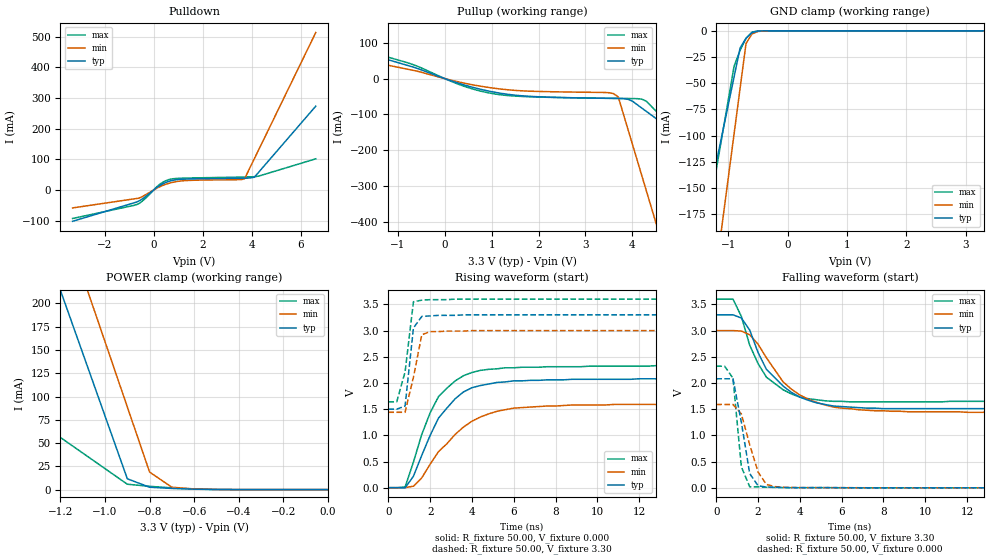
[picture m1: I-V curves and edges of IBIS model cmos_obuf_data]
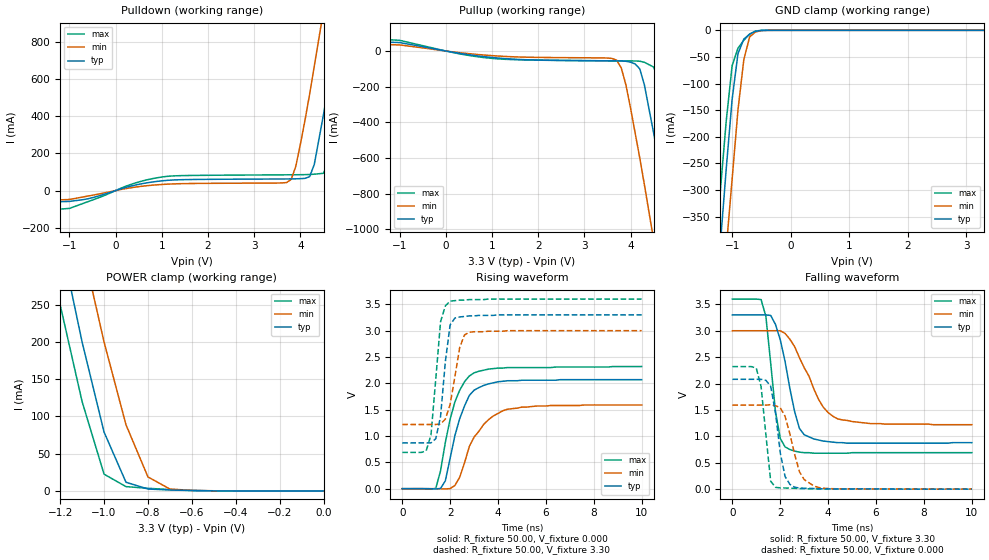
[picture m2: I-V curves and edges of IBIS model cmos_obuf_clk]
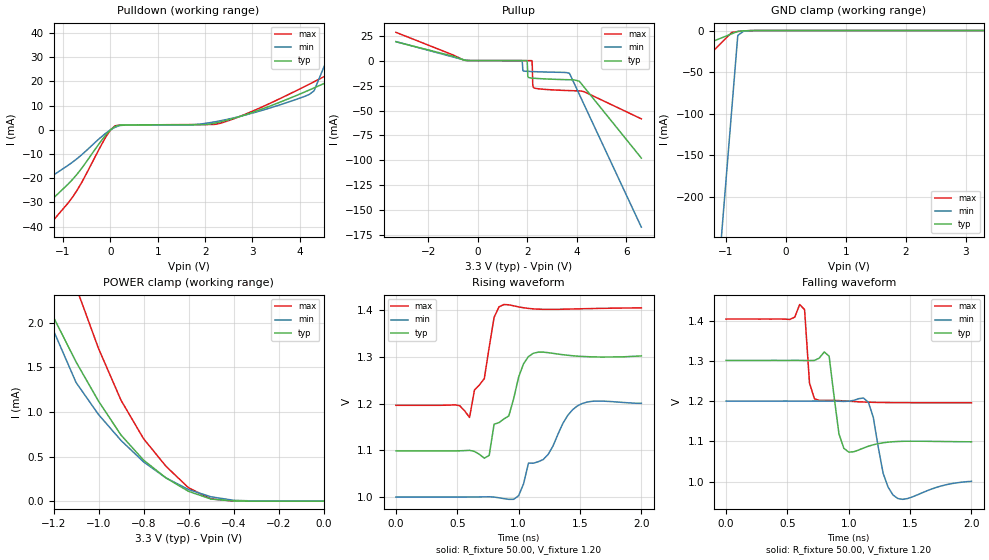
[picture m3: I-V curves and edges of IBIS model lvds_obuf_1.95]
| TEXAS INSTRUMENTS INCORPORATED
| High Performance Analog Group
| IBIS Model for ADS5545/46/47/25/27 series of A/D converters
| This file provides unique models under the [Model Selector] for each
| load condition.
| For operation at a specific load condition, select the appropriate model
|after each [Model Selector] keyword.
[IBIS ver]   3.2
[File name]   ads554x.ibs
[File Rev]   0
[Date]   17 Jul 2006
[Source]   Data created from TI-SPICE simulations
[Disclaimer] Property of Texas Instruments Incorporated.
   Unauthorized reproduction and/or distribution is strictly
   protected under copyright law. Created 2006, (C) Copyright
   2006, Texas Instruments Incorporated, All Rights Reserved
   UNLESS THERE IS A SIGNED, WRITTEN AGREEMENT TO THE CONTRARY,
   TEXAS INSTRUMENTS (TI) IS PROVIDING THE IBIS MODELS AND
   WITHOUT ANY WARRANTY, EXPRESSED OR IMPLIED. TI assumes no
   liability for: 1) the accuracy of the IBIS models provided to
   your company; 2) the proper functioning of these IBIS Models
   in your design or for any resulting applications; or 3)
   infringement of patents, copyrights or intellectual property
   rights resulting from your use of these IBIS models. TI
   provides IBIS Models as a service to our customers. You and
   your company shall not distribute, sell or give these models
   to anyone else without prior written permission from TI.
   TI reserves the right to make changes to our products or
   to discontinue any semiconductor product or service
   without notice, and advises our customers to obtain the
   latest version of relevant information to verify, before
   placing orders, that the information being relied on is
   current.
   Please be aware that your receipt and use of the IBIS
   information provided shall serve as acceptance of these
   terms and conditions.  If you do not accept these terms,
   you should return or destroy the IBIS models and any
   other accompanying information immediately.
[Notes]   This file contains IBIS Model of various buffers of
   ADS5545/46/47/25/27 series of A/D converters
[Copyright]   Property of Texas Instruments Incorporated. Unauthorised
   reproduction and/or distribution is strictly prohibited. This
   product is protected under copyright law and trade secret law
   as an unpublished work. Created 2000,(C) Copyright 2000,Texas
   Instruments Inc., All Rights Reserved.These commodities are
   under the U.S. Government distribution license control.As
   such,they are not to be re-exported without the prior approval
   of the U.S. Department of Commerce.
|   Component ADS554X
[Component]   ADS554X
[Manufacturer]   Texas Instruments
[Package]
| variable   typ   min   max
R_pkg   0.438   0.327   0.55
L_pkg   1.442nH   1.022nH   1.87nH
C_pkg   0.13pF   0.08390pF   0.201pF
[Pin]   signal_name   model_name   R_pin   L_pin   C_pin
|   (ohms)   (nH)   (pF)
1   DRGND   GND
2   DRVDD   POWER
3   OVR   cmos_obuf_data
4   CLKOUTM   clockoutm
5   CLKOUTP   clockoutp
|6   DFS   dummy
|7   OE   dummy
8   AVDD   POWER
9   AGND   POWER
10   CLKP   input
11   CLKM   input
12   AGND   GND
|13   VCMOUT / REFIN   dummy
14   AGND   GND
|15   INP   dummy
|16   INM   dummy
17   AGND   GND
18   AVDD   POWER
19   AGND   GND
20   AVDD   POWER
|21   IREF   dummy
22   AVDD   POWER
|23   MODE   dummy
24   AVDD   POWER
25   AGND   GND
26   AVDD   POWER
|27   SEN   dummy
|28   SDATA   dummy
|29   SCLK   dummy
|30   RESET   dummy
31   NC   NC
32   NC   NC
33   D0_D1M/D0   dataoutput
34   D0_D1P/D1   dataoutput
35   DRVDD   POWER
36   DRGND   GND
37   D2_D3M/D2   dataoutput
38   D2_D3P/D3   dataoutput
39   D4_D5M/D4   dataoutput
40   D4_D5P/D5   dataoutput
41   D6_D7M/D6   dataoutput
42   D6_D7P/D7   dataoutput
43   D8_D9M/D8   dataoutput
44   D8_D9P/D9   dataoutput
45   D10_D11M/D10   dataoutput
46   D10_D11P/D11   dataoutput
47   D12_D13M/D12   dataoutput
48   D12_D13P/D13   dataoutput
[Diff Pin]   inv_pin   vdiff   tdelay_typ   tdelay_min   tdelay_max
  4   5   350mV   0   0   0
  10   11   350mV   0   0   0
  34   33   350mV   0   0   0
  38   37   350mV   0   0   0
  40   39   350mV   0   0   0
  42   41   350mV   0   0   0
  44   43   350mV   0   0   0
  46   45   350mV   0   0   0
  48   47   350mV   0   0   0
[Series Pin Mapping]  pin_2   model_name   function_table_group
  4   5   series_res_166   1
  4   5   series_res_200   2
  4   5   series_res_333   3
  10   11   series_cap
  34   33   series_res_166   1
  34   33   series_res_200   2
  34   33   series_res_333   3
  38   37   series_res_166   1
  38   37   series_res_200   2
  38   37   series_res_333   3
  40   39   series_res_166   1
  40   39   series_res_200   2
  40   39   series_res_333   3
  42   41   series_res_166   1
  42   41   series_res_200   2
  42   41   series_res_333   3
  44   43   series_res_166   1
  44   43   series_res_200   2
  44   43   series_res_333   3
  46   45   series_res_166   1
  46   45   series_res_200   2
  46   45   series_res_333   3
  48   47   series_res_166   1
  48   47   series_res_200   2
  48   47   series_res_333   3
[Series Switch Groups]
| Following represent all possible switching combinations for 5 series elements
Off 1 2 3  /
Off 1 2 /
Off 2 3 /
Off 1 3 /
Off 1 /
Off 2 /
Off 3 /
On 1 2 3  /
[Model Selector] clockoutp
|The clock output can be in lvds mode or cmos mode. In lvds mode the
|clock signal ia a differential signal between pins CLKOUTP and CLKOUTM
|and in cmos mode its a single ended signal at pin CLKOUTP only.
|Note that the model for cmos buffer is different for data and clock output
|buffers whereas the model for the lvds buffer is the same
|  Model name   Description
cmos_obuf_clk   CMOS tri-state buffer
lvds_obuf_1.95   LVDS tri-state buffer with current setting 1.95mA
lvds_obuf_2.5   LVDS tri-state buffer with current setting 2.5mA
lvds_obuf_3.5   LVDS tri-state buffer with current setting 3.5mA
lvds_obuf_3.9   LVDS tri-state buffer with current setting 3.9mA
lvds_obuf_4.5   LVDS tri-state buffer with current setting 4.5mA
lvds_obuf_5.0   LVDS tri-state buffer with current setting 5.0mA
lvds_obuf_7.0   LVDS tri-state buffer with current setting 7.0mA
lvds_obuf_9.0   LVDS tri-state buffer with current setting 9.0mA
[Model Selector] clockoutm
|When the clock is output in the cmos mode, CLOCKOUTM is disabled. In the
|lvds mode the clock output is a differential signal between pins CLKOUTP
|and CLKOUTM.
|  Model name   Description
lvds_obuf_1.95   LVDS tri-state buffer with current setting 1.95mA
lvds_obuf_2.5   LVDS tri-state buffer with current setting 2.5mA
lvds_obuf_3.5   LVDS tri-state buffer with current setting 3.5mA
lvds_obuf_3.9   LVDS tri-state buffer with current setting 3.9mA
lvds_obuf_4.5   LVDS tri-state buffer with current setting 4.5mA
lvds_obuf_5.0   LVDS tri-state buffer with current setting 5.0mA
lvds_obuf_7.0   LVDS tri-state buffer with current setting 7.0mA
lvds_obuf_9.0   LVDS tri-state buffer with current setting 9.0mA
[Model Selector] dataoutput
|Note that the model for cmos buffer is different for data and clock output
|buffers whereas lvds buffer is the same
|  Model name
cmos_obuf_data   CMOS tri-state buffer
lvds_obuf_1.95   LVDS tri-state buffer with current setting 1.95mA
lvds_obuf_2.5   LVDS tri-state buffer with current setting 2.5mA
lvds_obuf_3.5   LVDS tri-state buffer with current setting 3.5mA
lvds_obuf_3.9   LVDS tri-state buffer with current setting 3.9mA
lvds_obuf_4.5   LVDS tri-state buffer with current setting 4.5mA
lvds_obuf_5.0   LVDS tri-state buffer with current setting 5.0mA
lvds_obuf_7.0   LVDS tri-state buffer with current setting 7.0mA
lvds_obuf_9.0   LVDS tri-state buffer with current setting 9.0mA
|   Model series_cap
[Model]   series_cap
Model_type   Series
C_comp   2.00pF   2.00pF   2.00pF
[Temperature Range]   27.00   125.00   -40.00
[Voltage Range]   3.30V   3.00V   3.60V
[C Series]   6.42pF   5.44pF   7.4pF
| End [Model] series_cap
|   Model series_res_166
[Model]   series_res_166
Model_type  Series_switch
C_comp   0.0F   NA   NA
[Temperature Range]   27   125   -40.0
[Voltage Range]   3.3000V   3.0000V   3.6000V
[On]
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[Off]
[R Series]   1.0000M   1.0000M   1.0000M
|End [Model]  series_res_166
|   Model series_res_200
[Model]   series_res_200
Model_type  Series_switch
C_comp   0.0F   NA   NA
[Temperature Range]   27   125   -40.0
[Voltage Range]   3.3000V   3.0000V   3.6000V
[On]
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[Off]
[R Series]   1.0000M   1.0000M   1.0000M
|End [Model]  series_res_200
|   Model series_res_333
[Model]   series_res_333
Model_type  Series_switch
C_comp   0.0F   NA   NA
[Temperature Range]   27   125   -40.0
[Voltage Range]   3.3000V   3.0000V   3.6000V
[On]
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[Off]
[R Series]   1.0000M   1.0000M   1.0000M
|End [Model]  series_res_333
| End [Component] ADS554X
| Models and submodels in the file (15): cmos_obuf_data (3-state), cmos_obuf_clk (3-state), lvds_obuf_1.95 (3-state), lvds_obuf_2.5 (3-state), lvds_obuf_3.5 (3-state), lvds_obuf_3.9 (3-state), lvds_obuf_4.5 (3-state), lvds_obuf_5.0 (3-state), lvds_obuf_7.0 (3-state), lvds_obuf_9.0 (3-state), input (Terminator), series_cap (Series), series_res_166 (Series_switch), series_res_200 (Series_switch), series_res_333 (Series_switch)
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|   Model cmos_obuf_data
[Model]   cmos_obuf_data
Model_type   3-state
Polarity   Non-Inverting
Enable   Active-High
Vmeas =   1.6000V
C_comp   1.00pF   1.00pF   1.00pF
[Temperature Range]   27.00   125   -40.00
[Voltage Range]   3.30V   3.00V   3.60V
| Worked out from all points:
|   slope of the pulldown table from 0 to 0.495 V, typ, clamps not added: 20.1 ohm
|   slope of the pullup table from 0 to 0.495 V, typ, clamps not added: 23.9 ohm
|   GND clamp passes 1 mA (typ) near -0.55 V on its own axis
|   POWER clamp passes 1 mA (typ) near -0.67 V on its own axis
|   rising waveform, R_fixture 50.00, V_fixture 0.000: 20-80 % time 1.72ns typ, 2.25ns min, 1.51ns max; typ from 0.001 V to 2.08 V
|   rising waveform, R_fixture 50.00, V_fixture 3.30: 20-80 % time 290ps typ, 499ps min, 423ps max; typ from 1.5 V to 3.3 V
|   falling waveform, R_fixture 50.00, V_fixture 3.30: 20-80 % time 1.8ns typ, 2.01ns min, 1.41ns max; typ from 3.3 V to 1.5 V
|   falling waveform, R_fixture 50.00, V_fixture 0.000: 20-80 % time 540ps typ, 692ps min, 329ps max; typ from 2.08 V to 0.002 V
[Pulldown]
| voltage   I(typ)   I(min)   I(max)
-3.3V     -102.3mA   -58.64mA   -93.08mA
-700mV    -39.68mA   -27.96mA   -48.04mA
-400mV    -25.64mA   -18.92mA   -32.04mA
100mV     6.34mA     4.54mA     8.27mA
300mV     16.89mA    12.43mA    21.39mA
700mV     30.05mA    23.46mA    35.49mA
1.3V      35.51mA    30.57mA    38.67mA
3.4V      38.09mA    33.52mA    41.69mA
3.7V      38.41mA    36.24mA    42.21mA
4.1V      41.55mA    102.1mA    43.3mA
4.3V      60.11mA    135.1mA    45.75mA
6.6V      273.5mA    513.9mA    101.6mA
[Pullup]
| voltage   I(typ)   I(min)   I(max)
-3.3V     132.6mA    93.64mA    138.3mA
-800mV    37.07mA    26.39mA    44.56mA
300mV     -13.08mA   -9.35mA    -16.01mA
900mV     -33.73mA   -24.03mA   -38.84mA
1.8V      -49.37mA   -35.03mA   -50.61mA
3.6V      -55.21mA   -41.92mA   -55.11mA
3.7V      -55.38mA   -51.34mA   -55.26mA
3.9V      -57.49mA   -138.8mA   -55.55mA
4.2V      -82.07mA   -270mA     -57.21mA
4.5V      -110.8mA   -401.2mA   -90.07mA
4.7V      -130mA     -488.6mA   -116.8mA
6.6V      -312mA     -1.32A     -371.3mA
[GND_clamp]
| voltage   I(typ)   I(min)   I(max)
-3.3V     -700mA     -1.13A     -825.4mA
-1.5V     -207.9mA   -356.3mA   -231.6mA
-1.4V     -180.6mA   -313.3mA   -198.6mA
-1.3V     -153.2mA   -270.3mA   -165.6mA
-1.1V     -98.53mA   -184.2mA   -99.65mA
-900mV    -43.85mA   -98.22mA   -33.67mA
-800mV    -16.51mA   -55.21mA   -18.65mA
-700mV    -7.1mA     -12.2mA    -7.18mA
-600mV    -1.83mA    -3.02mA    -1.24mA
-500mV    -210uA     -620uA     -74.65uA
-400mV    -14.42uA   -86.02uA   -2.09uA
3.3V      97.24pA    4.02uA     37.8pA
[POWER_clamp]
| voltage   I(typ)   I(min)   I(max)
-3.3V     1.631A     1.769A     407.6mA
-2.1V     821.4mA    929.1mA    206.7mA
-1.2V     214.1mA    298.9mA    56.01mA
-1.1V     146.6mA    228.9mA    39.27mA
-1V       79.1mA     158.9mA    22.53mA
-900mV    11.62mA    88.84mA    5.79mA
-800mV    2.56mA     18.82mA    3.53mA
-700mV    1.26mA     2.53mA     1.84mA
-600mV    480uA      710uA      650uA
-500mV    92.01uA    210uA      96.98uA
0V        97.24pA    6.35nA     47.29pA
[Ramp]
| variable   typ   min   max
dV/dt_r   1.25/1.60n   0.96/2.13n   1.39/1.45n
dV/dt_f   1.08/1.72n   0.93/1.89n   1.18/1.38n
R_load = 50.00
[Rising Waveform]
R_fixture = 50.00
V_fixture = 0.000
V_fixture_min = 0.000
V_fixture_max = 0.000
| time   V(typ)   V(min)   V(max)
0s        1.45mV     1.26mV     1.57mV
800ps     -2.01mV    1.79mV     14.11mV
1.2ns     220mV      30.5mV     490mV
1.6ns     620mV      190mV      1.02V
2.4ns     1.33V      690mV      1.74V
3.2ns     1.7V       1.02V      2.04V
4ns       1.91V      1.27V      2.2V
5.2ns     2.01V      1.46V      2.27V
7.6ns     2.06V      1.56V      2.31V
20ns      2.08V      1.6V       2.32V
[Rising Waveform]
R_fixture = 50.00
V_fixture = 3.30
V_fixture_min = 3.00
V_fixture_max = 3.60
| time   V(typ)   V(min)   V(max)
0s        1.5V       1.44V      1.64V
400ps     1.5V       1.44V      1.64V
800ps     1.56V      1.44V      2.21V
1.2ns     3.05V      2.11V      3.55V
1.6ns     3.27V      2.92V      3.58V
2ns       3.28V      2.98V      3.59V
3.6ns     3.3V       2.99V      3.6V
4ns       3.3V       3V         3.6V
20ns      3.3V       3V         3.6V
[Falling Waveform]
R_fixture = 50.00
V_fixture = 3.30
V_fixture_min = 3.00
V_fixture_max = 3.60
| time   V(typ)   V(min)   V(max)
0s        3.3V       3V         3.6V
800ps     3.3V       3V         3.6V
1.2ns     3.24V      2.99V      3.27V
1.6ns     3.01V      2.92V      2.72V
2.4ns     2.26V      2.48V      2.11V
3.2ns     1.94V      2.02V      1.87V
4ns       1.73V      1.77V      1.73V
5.6ns     1.56V      1.54V      1.65V
7.6ns     1.52V      1.47V      1.64V
20ns      1.5V       1.44V      1.64V
[Falling Waveform]
R_fixture = 50.00
V_fixture = 0.000
V_fixture_min = 0.000
V_fixture_max = 0.000
| time   V(typ)   V(min)   V(max)
0s        2.08V      1.59V      2.32V
400ps     2.08V      1.59V      2.32V
800ps     2.08V      1.59V      2.09V
1.2ns     1.25V      1.41V      400mV
1.6ns     270mV      820mV      19.08mV
2ns       39.06mV    300mV      16.29mV
2.4ns     14.15mV    63.42mV    10.45mV
2.8ns     10.42mV    22.85mV    6.6mV
4.4ns     2.33mV     2.75mV     2.56mV
20ns      1.67mV     1.42mV     1.85mV
|   Model cmos_obuf_clk
[Model]   cmos_obuf_clk
Model_type   3-state
Polarity   Non-Inverting
Enable   Active-High
Vmeas =   1.6000V
C_comp   1.00pF   1.00pF   1.00pF
[Temperature Range]   27.00   0.12k   -40.00
[Voltage Range]   3.30V   3.00V   3.60V
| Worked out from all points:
|   slope of the pulldown table from 0 to 0.495 V, typ, clamps not added: 14.9 ohm
|   slope of the pullup table from 0 to 0.495 V, typ, clamps not added: 23.9 ohm
|   GND clamp passes 1 mA (typ) near -0.55 V on its own axis
|   POWER clamp passes 1 mA (typ) near -0.67 V on its own axis
|   rising waveform, R_fixture 50.00, V_fixture 0.000: 20-80 % time 763ps typ, 1.04ns min, 741ps max; typ from 0.002 V to 2.07 V
|   rising waveform, R_fixture 50.00, V_fixture 3.30: 20-80 % time 322ps typ, 404ps min, 325ps max; typ from 0.87 V to 3.3 V
|   falling waveform, R_fixture 50.00, V_fixture 3.30: 20-80 % time 659ps typ, 1.11ns min, 420ps max; typ from 3.3 V to 0.88 V
|   falling waveform, R_fixture 50.00, V_fixture 0.000: 20-80 % time 408ps typ, 550ps min, 310ps max; typ from 2.08 V to -0.001 V
[Pulldown]
| voltage   I(typ)   I(min)   I(max)
-3.3V     -91.43mA   -94.62mA   -187.1mA
-1V       -58.73mA   -48.32mA   -96.41mA
1V        52.25mA    32.74mA    72.89mA
3.7V      62.47mA    43.03mA    84.85mA
3.9V      63.2mA     130mA      85.22mA
4.2V      75.01mA    520mA      86.64mA
4.5V      410mA      970mA      93.03mA
4.7V      710mA      1.28A      210mA
4.9V      1.02A      1.59A      490mA
5.1V      1.33A      1.91A      800mA
5.3V      1.65A      2.23A      1.12A
6.6V      3.75A      4.31A      3.23A
[Pullup]
| voltage   I(typ)   I(min)   I(max)
-3.3V     93.69mA    67.07mA    120.5mA
1V        -36.4mA    -25.92mA   -41.37mA
3.7V      -55.38mA   -51.34mA   -55.26mA
3.9V      -57.49mA   -190mA     -55.55mA
4.2V      -100mA     -600mA     -57.21mA
4.3V      -190mA     -750mA     -63.29mA
4.5V      -460mA     -1.06A     -90.07mA
4.7V      -750mA     -1.37A     -230mA
4.9V      -1.06A     -1.67A     -510mA
5.1V      -1.37A     -1.99A     -810mA
5.3V      -1.68A     -2.3A      -1.12A
6.6V      -3.73A     -4.35A     -3.17A
[GND_clamp]
| voltage   I(typ)   I(min)   I(max)
-3.3V     -3.73A     -3.87A     -3.65A
-1.3V     -550mA     -700mA     -450mA
-1.2V     -400mA     -560mA     -300mA
-1.1V     -260mA     -410mA     -170mA
-1V       -130mA     -280mA     -66.66mA
-900mV    -43.85mA   -150mA     -33.67mA
-800mV    -16.51mA   -55.21mA   -18.65mA
-700mV    -7.1mA     -12.2mA    -7.18mA
-600mV    -1.83mA    -3.02mA    -1.24mA
-400mV    -14.42uA   -86.02uA   -2.09uA
3.3V      97.24pA    4.02uA     37.8pA
[POWER_clamp]
| voltage   I(typ)   I(min)   I(max)
-3.3V     3.6A       3.72A      3.53A
-1.3V     480mA      620mA      400mA
-1.2V     340mA      480mA      250mA
-1.1V     200mA      330mA      120mA
-1V       79.1mA     200mA      22.53mA
-900mV    11.62mA    88.84mA    5.79mA
-800mV    2.56mA     18.82mA    3.53mA
-700mV    1.26mA     2.53mA     1.84mA
-500mV    92.01uA    210uA      96.98uA
0V        97.24pA    6.35nA     47.29pA
[Ramp]
| variable   typ   min   max
dV/dt_r   1.24/0.76n   0.95/1.03n   1.39/0.73n
dV/dt_f   1.45/0.65n   1.06/1.09n   1.74/0.38n
R_load = 50.00
[Rising Waveform]
R_fixture = 50.00
V_fixture = 0.000
V_fixture_min = 0.000
V_fixture_max = 0.000
| time   V(typ)   V(min)   V(max)
0s        1.52mV     1.3mV      1.64mV
1.4ns     -3.81mV    1.52mV     7.29mV
1.6ns     6.17mV     -670uV     340mV
1.8ns     150mV      -4.1mV     880mV
2.2ns     1.01V      62.41mV    1.65V
2.6ns     1.57V      490mV      2.03V
3ns       1.87V      980mV      2.2V
3.6ns     1.99V      1.31V      2.27V
4.4ns     2.05V      1.51V      2.3V
10ns      2.07V      1.59V      2.32V
[Rising Waveform]
R_fixture = 50.00
V_fixture = 3.30
V_fixture_min = 3.00
V_fixture_max = 3.60
| time   V(typ)   V(min)   V(max)
0s        870mV      1.22V      690mV
1ns       870mV      1.22V      720mV
1.2ns     870mV      1.22V      1.02V
1.4ns     950mV      1.22V      2.08V
1.6ns     1.37V      1.23V      3.17V
1.8ns     2.41V      1.32V      3.47V
2ns       3.11V      1.6V       3.56V
2.4ns     3.26V      2.68V      3.58V
2.8ns     3.28V      2.97V      3.59V
10ns      3.3V       3V         3.6V
[Falling Waveform]
R_fixture = 50.00
V_fixture = 3.30
V_fixture_min = 3.00
V_fixture_max = 3.60
| time   V(typ)   V(min)   V(max)
0s        3.3V       3V         3.6V
1.2ns     3.3V       3V         3.59V
1.4ns     3.3V       3V         3.27V
1.8ns     3.12V      3V         1.47V
2ns       2.83V      3V         960mV
2.2ns     2.42V      2.95V      800mV
2.8ns     1.15V      2.49V      700mV
3.4ns     950mV      1.9V       680mV
4.4ns     880mV      1.33V      680mV
10ns      880mV      1.22V      690mV
[Falling Waveform]
R_fixture = 50.00
V_fixture = 0.000
V_fixture_min = 0.000
V_fixture_max = 0.000
| time   V(typ)   V(min)   V(max)
0s        2.08V      1.59V      2.32V
1ns       2.08V      1.59V      2.29V
1.2ns     2.08V      1.59V      1.94V
1.6ns     1.95V      1.6V       150mV
1.8ns     1.45V      1.58V      33.89mV
2.2ns     240mV      1.38V      20.65mV
2.6ns     36.65mV    660mV      14.78mV
3ns       15.67mV    180mV      8.05mV
3.6ns     8.31mV     30.89mV    3.01mV
10ns      -600uV     77.02uV    -990uV
|   Model lvds_obuf_1.95
[Model]   lvds_obuf_1.95
Model_type   3-state
Polarity   Non-Inverting
Enable   Active-High
Vmeas =   1.2000V
Cref =   5.0000pF
Rref = 50.0000
Vref =   1.2000V
C_comp   2.13pF   1.93pF   2.34pF
[Temperature Range]   27.00   125   -40.00
[Voltage Range]   3.30V   3.00V   3.60V
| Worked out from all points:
|   slope of the pulldown table from 0 to 0.495 V, typ, clamps not added: 241 ohm
|   GND clamp passes 1 mA (typ) near -0.79 V on its own axis
|   POWER clamp passes 1 mA (typ) near -0.97 V on its own axis
|   rising waveform, R_fixture 50.00, V_fixture 1.20: 20-80 % time 216ps typ, 316ps min, 113ps max; typ from 1.1 V to 1.3 V
|   falling waveform, R_fixture 50.00, V_fixture 1.20: 20-80 % time 50.7ps typ, 68.6ps min, 33.4ps max; typ from 1.3 V to 1.1 V
[Pulldown]
| voltage   I(typ)   I(min)   I(max)
-3.3V     -67mA      -46mA      -85.16mA
-2.1V     -44.8mA    -30.4mA    -57.8mA
-1.5V     -33.7mA    -22.6mA    -44.12mA
-800mV    -20.55mA   -13.41mA   -27.86mA
100mV     1.4mA      1.04mA     1.63mA
2.2V      2.7mA      3.25mA     2.2mA
3.6V      11.52mA    10.4mA     13.03mA
4.3V      17.26mA    16.04mA    19.8mA
4.9V      27.14mA    44.42mA    25.87mA
5.1V      46.05mA    53.88mA    28.1mA
5.5V      83.87mA    72.8mA     58.7mA
6.6V      187.9mA    124.8mA    177.2mA
[Pullup]
| voltage   I(typ)   I(min)   I(max)
-3.3V     18.96mA    19.1mA     28.4mA
-500mV    350uA      560uA      320uA
1.78V     19.31uA    7.043uA    37.05uA
1.82V     17.88uA    -9.814mA   34.71uA
1.98V     8.748uA    -10.66mA   25.27uA
2.02V     -15.71mA   -10.69mA   22.9uA
2.18V     -17.47mA   -10.94mA   1.972uA
2.22V     -17.55mA   -10.98mA   -24.66mA
2.26V     -17.63mA   -11.02mA   -27.08mA
3.7V      -19.14mA   -12.68mA   -30.04mA
4.1V      -20.7mA    -33.96mA   -30.36mA
6.6V      -97.7mA    -167mA     -58.37mA
[GND_clamp]
| voltage   I(typ)   I(min)   I(max)
-3.3V     -73.53mA   -2.228A    -176.7mA
-1.1V     -9.73mA    -272.6mA   -16.77mA
-1V       -6.83mA    -183.7mA   -9.5mA
-900mV    -3.93mA    -94.8mA    -2.23mA
-800mV    -1.03mA    -5.92mA    -1.19mA
-700mV    -450uA     -730uA     -490uA
3.3V      44.64pA    1.08uA     37.43pA
[POWER_clamp]
| voltage   I(typ)   I(min)   I(max)
-3.3V     247.8mA    491.9mA    558.7mA
-1.3V     2.62mA     3.21mA     3.99mA
-1.2V     2.06mA     1.91mA     3.16mA
-1.1V     1.56mA     1.33mA     2.4mA
-1V       1.12mA     970uA      1.71mA
-900mV    740uA      680uA      1.13mA
-800mV    460uA      440uA      700uA
-700mV    260uA      260uA      390uA
-600mV    110uA      130uA      150uA
-500mV    23.34uA    48.47uA    24.97uA
-400mV    2uA        9.55uA     1.31uA
0V        44.64pA    500pA      43.31pA
[Ramp]
| variable   typ   min   max
dV/dt_r   1.84/71.06p   1.61/0.12n   2.05/48.53p
dV/dt_f   1.15/91.14p   1.12/0.15n   1.20/59.63p
R_load = 1.00k
[Rising Waveform]
R_fixture = 50.00
V_fixture = 1.20
V_fixture_min = 1.10
V_fixture_max = 1.30
| time   V(typ)   V(min)   V(max)
0s        1.099V     999.8mV    1.196V
600ps     1.1V       999.9mV    1.17V
720ps     1.083V     1V         1.253V
760ps     1.089V     1V         1.32V
800ps     1.156V     999.7mV    1.385V
880ps     1.167V     996.4mV    1.412V
1ns       1.257V     1.003V     1.407V
1.12ns    1.308V     1.072V     1.403V
1.48ns    1.301V     1.195V     1.403V
2ns       1.302V     1.2V       1.405V
[Falling Waveform]
R_fixture = 50.00
V_fixture = 1.20
V_fixture_min = 1.10
V_fixture_max = 1.30
| time   V(typ)   V(min)   V(max)
0s        1.302V     1.2V       1.405V
600ps     1.302V     1.2V       1.441V
640ps     1.302V     1.2V       1.428V
680ps     1.301V     1.2V       1.245V
800ps     1.323V     1.2V       1.202V
1ns       1.073V     1.2V       1.2V
1.16ns    1.088V     1.197V     1.198V
1.28ns    1.097V     1.02V      1.197V
1.4ns     1.1V       957.6mV    1.196V
2ns       1.099V     1V         1.196V
